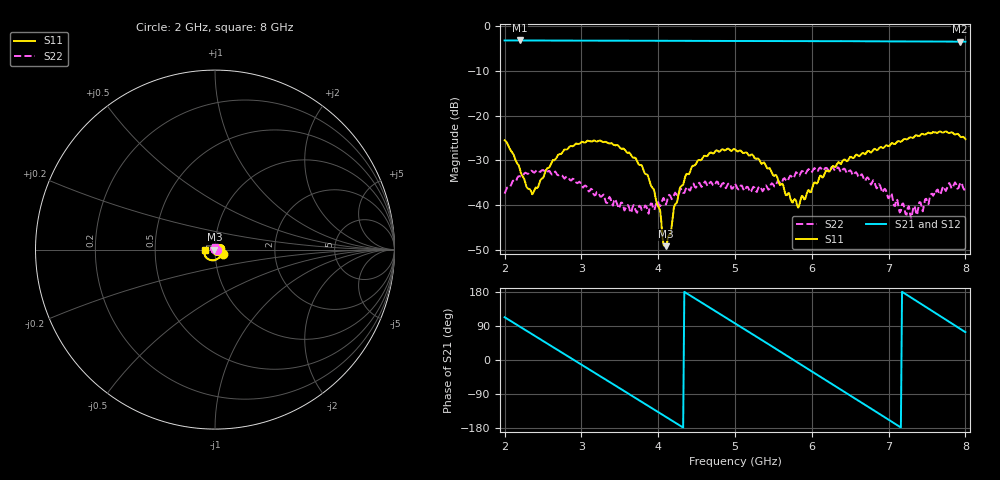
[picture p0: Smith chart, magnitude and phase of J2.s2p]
!Agilent Technologies,E8364B,MY43040699,A.07.50.67
!Agilent E8364B: A.07.50.67
!Date: Friday, June 06, 2025 05:51:00
!Correction: S11(Full 2 Port(1,2))
!S21(Full 2 Port(1,2))
!S12(Full 2 Port(1,2))
!S22(Full 2 Port(1,2))
!S2P File: Measurements: S11, S21, S12, S22:
# Hz S  dB  R 50
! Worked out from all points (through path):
!   401 points, 2 GHz to 8 GHz, reference 50 ohm
!   highest |S21| = -3.20 dB at 2.195 GHz (marker M1); lowest = -3.5 dB at 7.925 GHz (marker M2)
!   group delay of S21, straight-line fit = 351 ps
!   lowest |S11| = -49.2 dB at 4.1 GHz (marker M3), VSWR 1.01, Z = 49.7 - j0.124 ohm
!   |S11| at or under -10 dB: start of sweep to end of sweep
!   |S22| runs from -43.1 to -31.5 dB; largest |S21 - S12| = 0.0024
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2e9  -25.55 -30.4  -3.20 112.9  -3.20 112.9  -37.45 -3.7
2.195e9  -31.71 -35.0  -3.20 88.5  -3.20 88.5  -33.54 -34.2
2.375e9  -37.20 17.0  -3.21 66.0  -3.20 66.0  -32.69 -61.2
2.705e9  -28.66 41.3  -3.22 24.7  -3.21 24.7  -33.35 -107.3
3.005e9  -25.85 18.7  -3.24 -12.8  -3.23 -12.8  -35.81 -158.5
3.53e9  -27.44 -33.5  -3.26 -78.5  -3.25 -78.4  -39.49 123.3
3.845e9  -33.14 -69.6  -3.26 -118.0  -3.26 -117.9  -40.27 95.5
4.01e9  -40.62 -99.1  -3.27 -138.7  -3.26 -138.7  -40.04 89.7
4.1e9  -49.21 -159.0  -3.27 -150.1  -3.27 -150.0  -39.92 89.0
4.28e9  -36.38 77.0  -3.27 -172.7  -3.29 -172.6  -36.89 78.9
4.445e9  -31.23 50.7  -3.29 166.6  -3.29 166.6  -35.49 59.2
5e9  -27.52 -23.8  -3.32 96.7  -3.32 96.8  -35.22 -26.2
5.27e9  -29.66 -60.0  -3.33 62.6  -3.32 62.7  -36.90 -90.4
5.555e9  -34.08 -116.2  -3.33 26.6  -3.33 26.7  -34.63 -147.8
5.81e9  -40.19 151.8  -3.34 -5.7  -3.34 -5.7  -32.91 163.1
6.005e9  -36.27 90.5  -3.35 -30.5  -3.35 -30.4  -32.55 142.0
6.5e9  -29.23 5.4  -3.35 -93.5  -3.37 -93.5  -32.23 88.9
7.01e9  -26.81 -53.6  -3.40 -158.8  -3.40 -158.8  -38.31 72.8
7.265e9  -24.98 -82.7  -3.41 168.4  -3.41 168.4  -40.27 84.3
7.415e9  -24.33 -100.7  -3.42 149.1  -3.42 149.1  -39.40 99.9
7.925e9  -24.53 -169.8  -3.47 83.1  -3.44 83.2  -35.40 90.7
8e9  -25.25 179.6  -3.46 73.4  -3.45 73.4  -36.14 81.4
